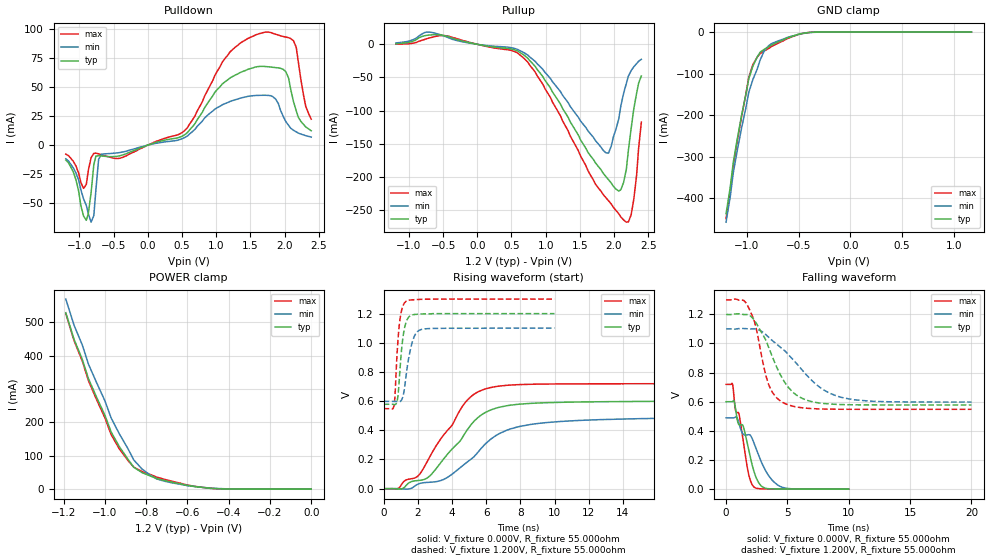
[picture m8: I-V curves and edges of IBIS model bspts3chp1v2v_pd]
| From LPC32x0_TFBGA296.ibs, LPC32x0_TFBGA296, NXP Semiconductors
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| |   Rev 0.20 IBIS Model Design Automation Generation   |
| |   N O N - S I L I C O N   C O R R E L A T E D   |
| |   This IBIS [Model] is pre-Beta tactical support   |
| |  Note: this IBIS [Model] contains clamp curves generated   |
| |   through simulation which should not be relied upon   |
| bspts3chp1v2v
|   Bidirectional Pad 1v2
|   3state Output
|   Plain Input
|   3ns Slew Rate control
|   CMOS
|   Programmable between
|   - (p1=0, p2=1) plain input
|   - (p1=0, p2=0) with Pull Up
|   - (p1=1, p2=1) with Pull Down
|   - (p1=1, p2=0) with Repeater
|   Characterized at Core 1.2V and I/O 1.2V
| Pull Down Mode (p1=1, p2=1)
[Model]   bspts3chp1v2v_pd | of bspts3chp1v2v
Model_type   I/O
Polarity   Non-Inverting
Enable   Active-Low
|  Reciever Thresholds
Vinl   = 0.36V
Vinh   = 0.84V
| AC Test Load Conditions
Vref   = 0
Cref   = 1.2e-11
Rref   = 1000000000
Vmeas   = 0.6
| [Process Range]   typical   min   max
| C_comp edge width   400.000ps   400.000ps   400.000ps
| C_comp Tstrobe   40.000fs   40.000fs   40.000fs
C_comp   2.969pF   2.762pF   3.249pF
[Temperature Range]   25   105   -20
[Voltage Range]   1.20V   1.10V   1.30V
[GND Clamp Reference]   0.00V   0.00V   0.00V
[Pulldown Reference]   0.00V   0.00V   0.00V
[POWER Clamp Reference]   1.20V   1.10V   1.30V
[Pullup Reference]   1.20V   1.10V   1.30V
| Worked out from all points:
|   slope of the pulldown table from 0 to 0.18 V, typ, clamps not added: 55.1 ohm
|   slope of the pullup table from 0 to 0.18 V, typ, clamps not added: 53.4 ohm
|   GND clamp passes 1 mA (typ) near -0.40 V on its own axis
|   POWER clamp passes 1 mA (typ) near -0.43 V on its own axis
|   rising waveform, V_fixture 0.000V, R_fixture 55.000ohm: 20-80 % time 2.49ns typ, 3.01ns min, 2.32ns max; typ from 0 V to 0.599 V
|   falling waveform, V_fixture 0.000V, R_fixture 55.000ohm: 20-80 % time 1.38ns typ, 2.14ns min, 1.03ns max; typ from 0.6 V to 0 V
|   rising waveform, V_fixture 1.200V, R_fixture 55.000ohm: 20-80 % time 291ps typ, 433ps min, 251ps max; typ from 0.578 V to 1.2 V
|   falling waveform, V_fixture 1.200V, R_fixture 55.000ohm: 20-80 % time 2.15ns typ, 3.59ns min, 1.25ns max; typ from 1.2 V to 0.578 V
[GND Clamp]
| ref voltage   0.00V   0.00V   0.00V
|   Voltage   I(typ)   I(min)   I(max)
-1.2V     -437mA     -457.3mA   -448.8mA
-1.16V    -374mA     -396.6mA   -383.9mA
-1.13V    -313.1mA   -338.2mA   -320.9mA
-1.05V    -200.5mA   -230.7mA   -202.9mA
-980mV    -111.6mA   -144.4mA   -108mA
-940mV    -81.38mA   -113.4mA   -77.56mA
-870mV    -48.14mA   -66.68mA   -51.43mA
-830mV    -41.13mA   -44.64mA   -45.15mA
-790mV    -35.75mA   -33.05mA   -39.64mA
-570mV    -10.72mA   -10.13mA   -11.97mA
-390mV    -634.3uA   -1.09mA    -536.4uA
1.17V     20.93uA    11.34uA    34.93uA
[Power Clamp]   | Vtable = Vcc - Vpad
| ref voltage   1.20V   1.10V   1.30V
|   Voltage   I(typ)   I(min)   I(max)
-1.19V    529.3mA    570.1mA    526.5mA
-1.15V    449.5mA    491.7mA    445.3mA
-1.11V    389.5mA    432.5mA    384.2mA
-1.08V    331.1mA    374.7mA    324.8mA
-1V       221.2mA    264.5mA    213.3mA
-970mV    171.4mA    213.2mA    163.4mA
-890mV    91.03mA    122.9mA    86.97mA
-860mV    65.37mA    87.22mA    65.76mA
-820mV    49.51mA    60.16mA    53.06mA
-750mV    32.08mA    30.86mA    36.26mA
-560mV    7.534mA    7.568mA    8.097mA
0V        20.95uA    11.19uA    35.02uA
[Pulldown]
| ref voltage   0.00V   0.00V   0.00V
|   Voltage   I(typ)   I(min)   I(max)
-1.2V     -12.9mA    -11.81mA   -7.732mA
-900mV    -64.77mA   -51.94mA   -33.88mA
-830mV    -40.99mA   -66.41mA   -10.77mA
-760mV    -9.399mA   -38.71mA   -6.922mA
-720mV    -9.108mA   -12.33mA   -7.471mA
-680mV    -9.342mA   -7.831mA   -8.122mA
500mV     7.667mA    5.475mA    10.77mA
1.2V      57.8mA     37.61mA    80.16mA
1.72V     67.75mA    42.98mA    97.43mA
2.02V     63.12mA    20.22mA    93.1mA
2.13V     37.64mA    12.84mA    90mA
2.39V     12.34mA    6.89mA     22.38mA
[Pullup]   | Vtable = Vcc - Vpad
| ref voltage   1.20V   1.10V   1.30V
|   Voltage   I(typ)   I(min)   I(max)
-1.19V    982.9uA    2.112mA    262.9uA
-710mV    13.91mA    18.44mA    9.272mA
-450mV    12.25mA    11.02mA    12.78mA
590mV     -9.985mA   -7.698mA   -13.1mA
960mV     -48.84mA   -37.98mA   -60.41mA
1.88V     -199.3mA   -163.7mA   -231.3mA
1.96V     -209.3mA   -153.4mA   -241mA
2.07V     -221.5mA   -112.3mA   -255.7mA
2.18V     -188.8mA   -59.17mA   -268.4mA
2.25V     -127.4mA   -39.92mA   -257.5mA
2.33V     -74.27mA   -29.16mA   -198.1mA
2.4V      -47.76mA   -22.65mA   -117.4mA
[Ramp]
R_load   = 55.000ohm
|   dV/dt(typ)   dV/dt(min)   dV/dt(max)
dV/dt_r   337.978mV/2.450ns   259.332mV/2.715ns   412.738mV/2.315ns
dV/dt_f   356.284mV/2.205ns   272.265mV/3.345ns   433.775mV/1.330ns
[Rising Waveform]  | cubic spline decimation from 4001 points
V_fixture   = 0.000V
R_fixture   = 55.000ohm
|   Time   V(typ)   V(min)   V(max)
0s        162.8nV    2.485uV    161.4nV
755ps     -1.211mV   314.8uV    -2.713mV
1.945ns   55.04mV    27.45mV    80.76mV
2.63ns    80.36mV    43.51mV    203.3mV
3.51ns    203.6mV    63.23mV    367.7mV
4.8ns     386.7mV    174.1mV    593.9mV
5.985ns   524.1mV    310.2mV    684.6mV
7.205ns   568.2mV    400.4mV    708mV
9.085ns   587.1mV    447.5mV    716.2mV
20ns      599.4mV    486.2mV    719.2mV
[Falling Waveform]  | cubic spline decimation from 2001 points
V_fixture   = 0.000V
R_fixture   = 55.000ohm
|   Time   V(typ)   V(min)   V(max)
0s        600.3mV    489.5mV    719.4mV
525ps     601.8mV    489.6mV    721.9mV
755ps     562.7mV    494.4mV    549mV
1.055ns   442.8mV    451.9mV    516.2mV
1.4ns     432.2mV    377.6mV    331.5mV
1.815ns   282.8mV    373.9mV    112.8mV
2.29ns    117.5mV    313.4mV    13.8mV
2.96ns    15.79mV    170.8mV    1.945mV
4.385ns   881.1uV    19.75mV    309.4uV
10ns      7.647uV    93.44uV    1.443uV
[Rising Waveform]  | cubic spline decimation from 2001 points
V_fixture   = 1.200V
V_fixture_min = 1.100V
V_fixture_max = 1.300V
R_fixture   = 55.000ohm
|   Time   V(typ)   V(min)   V(max)
0s        578.2mV    598.1mV    548.2mV
600ps     576.6mV    598.1mV    566.9mV
670ps     576mV      598.1mV    650.6mV
780ps     596.8mV    596.9mV    911.4mV
985ps     864.1mV    599mV      1.183V
1.15ns    1.054V     641.6mV    1.258V
1.33ns    1.146V     789.2mV    1.285V
1.7ns     1.191V     1.014V     1.294V
2.215ns   1.197V     1.091V     1.297V
10ns      1.199V     1.1V       1.299V
[Falling Waveform]  | cubic spline decimation from 4001 points
V_fixture   = 1.200V
V_fixture_min = 1.100V
V_fixture_max = 1.300V
R_fixture   = 55.000ohm
|   Time   V(typ)   V(min)   V(max)
0s        1.199V     1.1V       1.299V
1.4ns     1.199V     1.103V     1.297V
1.77ns    1.198V     1.101V     1.258V
2.4ns     1.148V     1.1V       1.124V
3.09ns    1.047V     1.072V     835.8mV
3.495ns   968.6mV    1.041V     713.5mV
4.845ns   725.4mV    945mV      586.2mV
6.505ns   612.9mV    788.9mV    556.1mV
9.36ns    581mV      631.2mV    548.6mV
20ns      578.2mV    598.1mV    548.2mV
